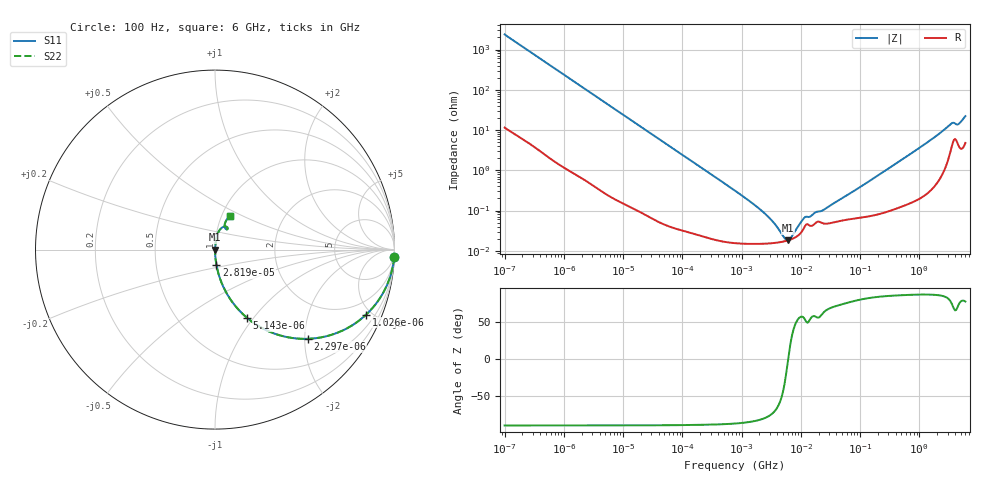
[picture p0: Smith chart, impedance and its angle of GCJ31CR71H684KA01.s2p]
!Murata Part Number: GCJ31CR71H684KA01
!These Parameters are Measured in Series Mode Connection
!Data Generated on Mar 13, 2026
!  o--ll--o
!Port1  Port2
!  o------o
!Operation Temp=25[degC], DC Bias Voltage=0[V]
!Freq. Start=100[Hz] Stop=6[GHz] 401[Steps]
# Hz S RI R 50
!Freq.(Hz) S11(Real) S11(Imag) S21(Real) S21(Imag) S12(Real) S12(Imag) S22(Real) S22(Imag)
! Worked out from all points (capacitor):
!   401 points, 100 Hz to 6 GHz, reference 50 ohm
!   read as one part in series: C = 673 nF near 109 Hz
!   lowest |Z| = 18.1 mohm at 6.075 MHz (marker M1)
!   series resonance near 6.121 MHz, so ESL is about 1 nH
!   S11 on the Smith chart (normalised r, x): 100 Hz: 1, -47; 1.026 kHz: 1.02, -4.64; 2.297 kHz: 1.01, -2.08; 5.143 kHz: 1.01, -0.93; 28.19 kHz: 1.00, -0.17; 6 GHz: 1.10, +0.43
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100  0.998 -0.0422  0.00199 0.0422  0.00199 0.0422  0.998 -0.0422
335  0.9798 -0.1382  0.0202 0.1382  0.0202 0.1382  0.9798 -0.1382
1026  0.8421 -0.3622  0.1579 0.3622  0.1579 0.3622  0.8421 -0.3622
2008  0.5848 -0.4901  0.4152 0.4901  0.4152 0.4901  0.5848 -0.4901
2297  0.519 -0.497  0.481 0.497  0.481 0.497  0.519 -0.497
5143  0.1793 -0.3809  0.8207 0.3809  0.8207 0.3809  0.1793 -0.3809
10066  0.0549 -0.2248  0.9451 0.2248  0.9451 0.2248  0.0549 -0.2248
28191  0.0079 -0.0847  0.9921 0.0847  0.9921 0.0847  0.0079 -0.0847
40335  0.00407 -0.0595  0.9959 0.0595  0.9959 0.0595  0.00407 -0.0595
774597  0.000164 -0.00311  0.9998 0.00311  0.9998 0.00311  0.000164 -0.00311
2481164  0.000151 -0.000824  0.9998 0.000824  0.9998 0.000824  0.000151 -0.000824
3549919  0.000156 -0.000458  0.9998 0.000458  0.9998 0.000458  0.000156 -0.000458
5311619  0.000172 -0.000114  0.9998 0.000114  0.9998 0.000114  0.000172 -0.000114
6075234  0.000181 -6e-06  0.9998 6e-06  0.9998 6e-06  0.000181 -6e-06
6948629  0.000194 0.000103  0.9998 -0.000103  0.9998 -0.000103  0.000194 0.000103
1.137099e7  0.000374 0.000536  0.9996 -0.000536  0.9996 -0.000536  0.000374 0.000536
1.555665e7  0.00042 0.00065  0.9996 -0.00065  0.9996 -0.00065  0.00042 0.00065
2.545746e7  0.000471 0.000979  0.9995 -0.000979  0.9995 -0.000979  0.000471 0.000979
3.124326e8  0.0011 0.0114  0.9989 -0.0114  0.9989 -0.0114  0.0011 0.0114
3.352442e9  0.0447 0.126  0.9553 -0.126  0.9553 -0.126  0.0447 0.126
4.586474e9  0.0552 0.1217  0.9448 -0.1217  0.9448 -0.1217  0.0552 0.1217
6e9  0.0845 0.1887  0.9155 -0.1887  0.9155 -0.1887  0.0845 0.1887
